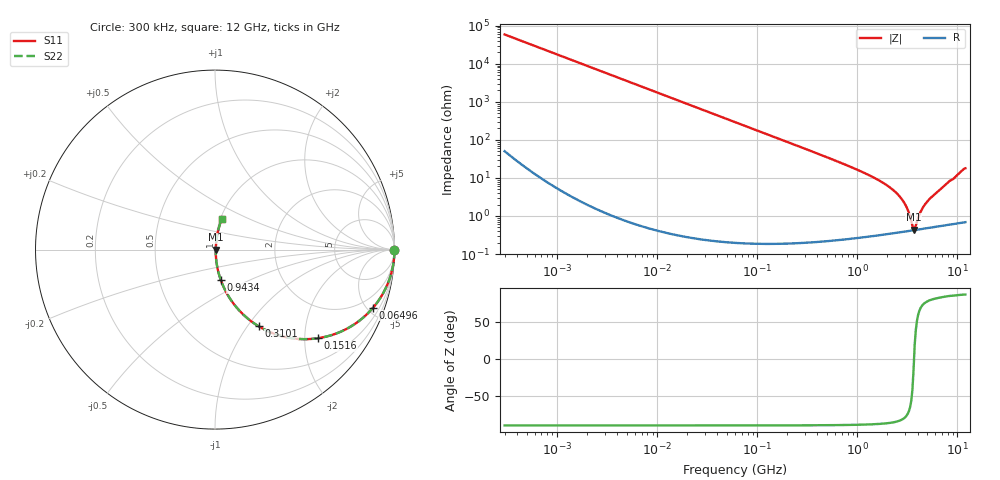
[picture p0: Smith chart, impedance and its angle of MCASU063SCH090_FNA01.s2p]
! MCASU063SCH090_FNA01  S-PARAMETER MODEL  ( Standard Model )
! Model Generated by TAIYO YUDEN Corporation (http://www.ty-top.com)
! Version 1.0
! TAIYO YUDEN Control No. 230609
! Copyright(c) 2023 TAIYO YUDEN CO.,LTD. All Rights Reserved.
! Product Description (link to TY-COMPAS)
! https://ds.yuden.co.jp/TYCOMPAS/or/detail?pn=MCASU063SCH090CFNA01&u=M
! Products Name : Multilayer Ceramic Capacitors
! Characteristics :
!  Capacitance : 9 [pF] , Rated Voltage : 50 [V] , TCC : CH / C0H
!  Case Size : 0.6 x 0.3 / 0.024 x 0.012 [mm/inch] , Thickness : 0.3 / 0.012 [mm/inch]
!  (Conditions: Temperature = 25 [degC] , DC Bias Voltage = 0 [V])
! External Node Assignments :
!  1  o---| |---o  2
! GND o---------o GND
! Frequency Range : 0.3MHz  -  12000MHz  [ 401 STEP ]
# MHZ S RI R 50
! Freq[MHz].  S11 Real  S11 Imag  S21 Real  S21 Imag  S12 Real  S12 Imag  S22 Real  S22 Imag
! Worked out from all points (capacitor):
!   401 points, 300 kHz to 12 GHz, reference 50 ohm
!   read as one part in series: C = 9 pF near 316.3 kHz
!   lowest |Z| = 435 mohm at 3.643 GHz (marker M1)
!   series resonance near 3.683 GHz, so ESL is about 210 pH
!   S11 on the Smith chart (normalised r, x): 300 kHz: open; 64.96 MHz: 1.00, -5.44; 151.6 MHz: 1.00, -2.33; 310.1 MHz: 1.00, -1.13; 943.4 MHz: 1.01, -0.35; 12 GHz: 1.01, +0.36
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0.3  1 -0.0017  4.33e-06 0.0017  4.33e-06 0.0017  1 -0.0017
1.769972  0.9999 -0.01  0.000102 0.01  0.000102 0.01  0.9999 -0.01
10.44266  0.9965 -0.0588  0.00349 0.0588  0.00349 0.0588  0.9965 -0.0588
26.39317  0.9782 -0.146  0.0218 0.146  0.0218 0.146  0.9782 -0.146
60  0.8965 -0.3042  0.1035 0.3042  0.1035 0.3042  0.8965 -0.3042
64.96309  0.8808 -0.3236  0.1192 0.3236  0.1192 0.3236  0.8808 -0.3236
99.25425  0.7599 -0.4266  0.2401 0.4266  0.2401 0.4266  0.7599 -0.4266
151.6462  0.5753 -0.4935  0.4247 0.4935  0.4247 0.4935  0.5753 -0.4935
310.0777  0.2436 -0.4275  0.7564 0.4275  0.7564 0.4275  0.2436 -0.4275
353.9943  0.1977 -0.3963  0.8023 0.3963  0.8023 0.3963  0.1977 -0.3963
943.3804  0.0321 -0.1691  0.9679 0.1691  0.9679 0.1691  0.0321 -0.1691
1519.776  0.0122 -0.0951  0.9878 0.0951  0.9878 0.0951  0.0122 -0.0951
2088.533  0.00664 -0.0569  0.9934 0.0569  0.9934 0.0569  0.00664 -0.0569
2514.07  0.00503 -0.0373  0.995 0.0373  0.995 0.0373  0.00503 -0.0373
2870.14  0.0044 -0.0241  0.9956 0.0241  0.9956 0.0241  0.0044 -0.0241
3190.978  0.00417 -0.0138  0.9958 0.0138  0.9958 0.0138  0.00417 -0.0138
3547.679  0.00416 -0.00368  0.9958 0.00368  0.9958 0.00368  0.00416 -0.00368
3642.919  0.00419 -0.00108  0.9958 0.00108  0.9958 0.00108  0.00419 -0.00108
3841.137  0.0043 0.00359  0.9957 -0.00359  0.9957 -0.00359  0.0043 0.00359
4385.161  0.00471 0.0137  0.9953 -0.0137  0.9953 -0.0137  0.00471 0.0137
5140.631  0.00547 0.0254  0.9945 -0.0254  0.9945 -0.0254  0.00547 0.0254
12000  0.0373 0.1712  0.9627 -0.1712  0.9627 -0.1712  0.0373 0.1712
